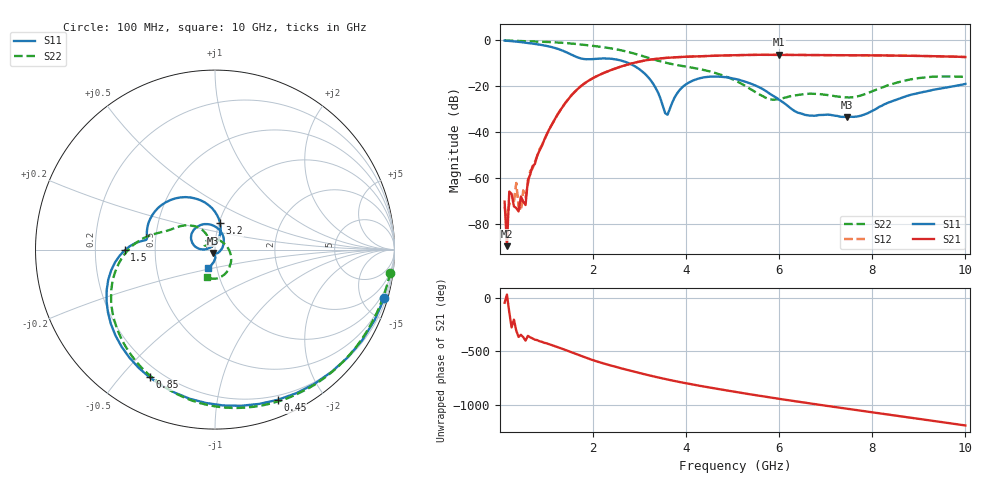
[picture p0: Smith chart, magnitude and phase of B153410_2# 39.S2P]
!  2-Port S-parameters saved by WinCal
! VAR MeasName=S-Parameters (CALIBRATED_DATA) read from VNA (N5245A)
! VAR MeasDate=2016-12-23 10:01:21
! VAR NAME=B153410_2# 39
! VAR FILENAME=B153410_2# 39.S2P
! VAR DATE=2016-12-23 10:01:21
! VAR PHYS_PORTS=1,2
# Hz S DB R 50
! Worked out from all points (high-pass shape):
!   199 points, 100 MHz to 10 GHz, reference 50 ohm
!   highest |S21| = -6.36 dB at 6 GHz (marker M1); lowest = -89.6 dB at 150 MHz (marker M2)
!   |S21| within 3 dB of the highest: 2.985 GHz to end of sweep
!   lowest |S11| = -33.4 dB at 7.45 GHz (marker M3), VSWR 1.04, Z = 49 - j1.84 ohm
!   |S11| at or under -10 dB: 2.763 GHz to end of sweep
!   |S22| runs from -25.9 to -0.1 dB; largest |S21 - S12| = 0.0017
!   S11 on the Smith chart (normalised r, x): 100 MHz: 0.48, -7.03; 450 MHz: 0.16, -1.49; 850 MHz: 0.15, -0.60; 1.5 GHz: 0.33, -0.00; 3.2 GHz: 1.01, +0.31; 10 GHz: 0.91, -0.19
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1e8  -0.16 -16.1  -70.24 -46.1  -72.55 -72.7  -0.13 -7.5
1.5e8  -0.25 -23.9  -89.62 29.7  -78.79 -117.5  -0.18 -11.0
2e8  -0.33 -31.5  -65.86 -133.4  -71.20 121.6  -0.22 -14.3
3e8  -0.53 -46.3  -72.31 156.8  -70.36 78.8  -0.28 -21.0
3.5e8  -0.62 -53.4  -73.03 54.7  -62.10 -36.0  -0.31 -24.3
4.5e8  -0.85 -67.3  -68.00 15.4  -74.24 32.0  -0.37 -30.9
5e8  -0.97 -74.0  -70.22 -6.6  -65.39 20.4  -0.39 -34.2
5.5e8  -1.09 -80.6  -71.71 -38.7  -68.47 -19.9  -0.43 -37.5
6e8  -1.21 -87.1  -60.87 5.4  -62.69 -8.6  -0.45 -40.8
8.5e8  -1.95 -117.2  -48.05 -44.6  -47.50 -44.6  -0.63 -57.1
1.5e9  -5.96 -179.5  -24.90 -141.4  -24.80 -141.3  -1.40 -98.6
1.75e9  -7.99 172.7  -19.83 177.3  -19.83 177.3  -1.91 -113.7
3.2e9  -16.47 79.2  -8.55 -1.4  -8.55 -1.3  -7.74 171.6
3.4e9  -22.98 71.7  -8.03 -21.6  -8.02 -21.5  -8.96 166.3
3.6e9  -32.44 138.7  -7.66 -40.7  -7.65 -40.7  -9.99 162.3
4.05e9  -18.52 169.2  -7.18 -79.8  -7.15 -79.8  -11.70 153.1
5.05e9  -16.83 102.7  -6.53 -155.2  -6.55 -155.2  -17.51 123.2
6e9  -25.93 26.5  -6.36 139.7  -6.37 139.7  -25.60 152.8
6.7e9  -32.81 -78.4  -6.43 94.6  -6.45 94.6  -23.31 143.4
7.45e9  -33.43 -118.3  -6.53 48.2  -6.54 48.2  -24.89 72.4
8.35e9  -27.13 -87.8  -6.67 -6.9  -6.66 -6.8  -19.51 -31.5
1e10  -19.04 -110.0  -7.33 -107.8  -7.33 -107.6  -16.01 -105.4
